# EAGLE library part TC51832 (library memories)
Pseudo static RAM 32Kx8 Toshiba
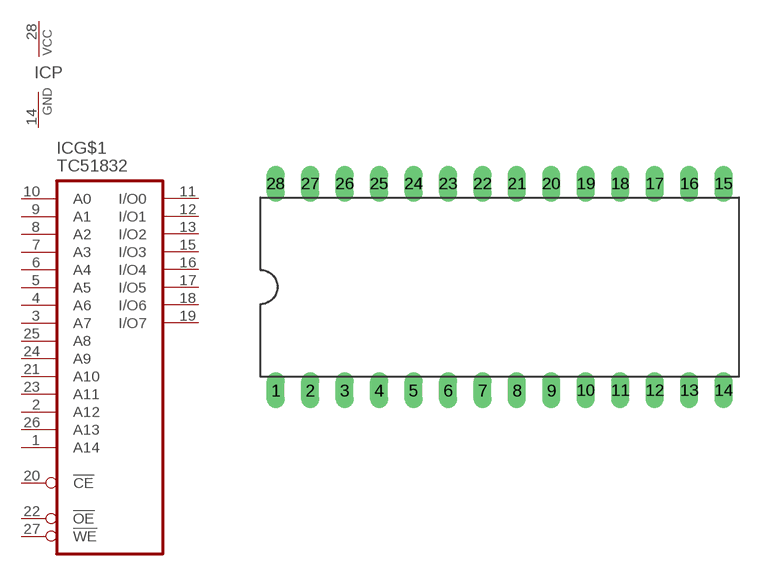
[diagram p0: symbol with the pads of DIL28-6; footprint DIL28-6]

Designator prefix IC; gates G$1=RAM32KX8 P=PWRN

## TC51832  [DIL28-6]
1  G$1:A14  in
2  G$1:A12  in
3  G$1:A7  in
4  G$1:A6  in
5  G$1:A5  in
6  G$1:A4  in
7  G$1:A3  in
8  G$1:A2  in
9  G$1:A1  in
10  G$1:A0  in
11  G$1:I/O0  hiz
12  G$1:I/O1  hiz
13  G$1:I/O2  hiz
14  P:GND  pwr
15  G$1:I/O3  hiz
16  G$1:I/O4  hiz
17  G$1:I/O5  hiz
18  G$1:I/O6  hiz
19  G$1:I/O7  hiz
20  G$1:!CE  in
21  G$1:A10  in
22  G$1:!OE  in
23  G$1:A11  in
24  G$1:A9  in
25  G$1:A8  in
26  G$1:A13  in
27  G$1:!WE  in
28  P:VCC  pwr

## Footprint DIL28-6 (pad centres in mm)
Dual In Line 0.6 inch
drill 0.813 long: 1 -16.51,-7.62; 2 -13.97,-7.62; 3 -11.43,-7.62; 4 -8.89,-7.62; 5 -6.35,-7.62; 6 -3.81,-7.62; 7 -1.27,-7.62; 8 1.27,-7.62; 9 3.81,-7.62; 10 6.35,-7.62; 11 8.89,-7.62; 12 11.43,-7.62; 13 13.97,-7.62; 14 16.51,-7.62; 15 16.51,7.62; 16 13.97,7.62; 17 11.43,7.62; 18 8.89,7.62; 19 6.35,7.62; 20 3.81,7.62; 21 1.27,7.62; 22 -1.27,7.62; 23 -3.81,7.62; 24 -6.35,7.62; 25 -8.89,7.62; 26 -11.43,7.62; 27 -13.97,7.62; 28 -16.51,7.62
